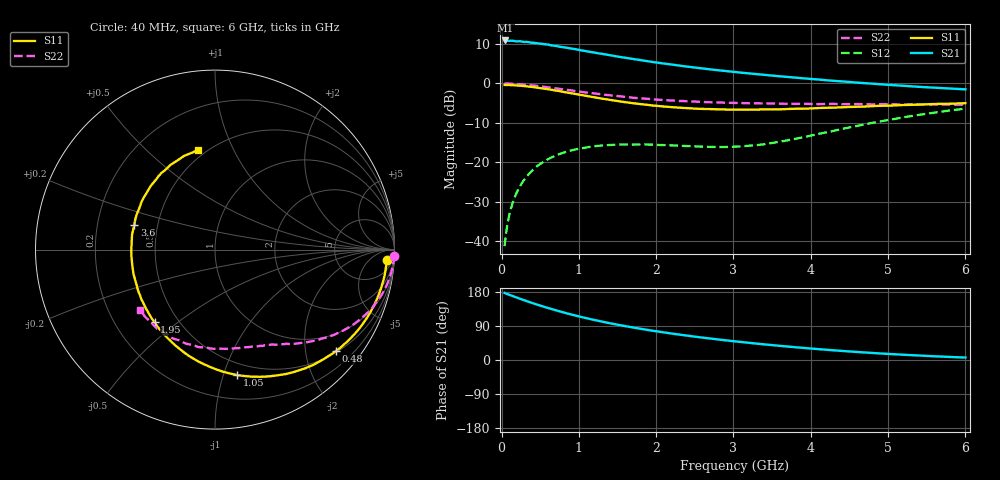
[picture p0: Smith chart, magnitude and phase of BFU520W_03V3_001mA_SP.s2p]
! Filename:  P:\Prog\Test\Noise\ATS_data\Testdata_Net\Run2\BFU520W_APM2013_06_A05_03p3V_001mA_SP_CM01_D.s2p
! Date/Time: Tue 26/Mar/2013 18:01:38
! BFU520W_APM2013_06_A05_03p3V_1to20mA_SP_CM01_Bias1_R.s2p
! MDIF S-parameter v. bias file
! BFU520W_APM2013_06_A05_03p3V_1to20mA_SP_CM01
! Date/time Tue Mar 19 16:47:37 2013
! bias mode 1
! bias variable = I_out
! VAR bias_var= 1
! VAR V_out= 3.3000
! VAR I_out= 1.0000
! VAR V_in= 0.7950
! VAR I_in= 0.0111
! Device data file deembeded for feedlines and parallel
! Original file: \Run2\BFU520W_APM2013_06_A05_03p3V_001mA_SP_CM01_R.s2p
! Feed-files: PR019V01_070313_Feed1.s2p, PR019V01_070313_Feed2.s2p
! Parallel-file: PR019V01_070313_Par.s2p
# MHz S MA R 50
!  Freq-MHz  S11-mag  S11-arg  S21-mag  S21-arg  S12-mag  S12-arg  S22-mag  S22-arg
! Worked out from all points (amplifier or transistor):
!   98 points, 40 MHz to 6 GHz, reference 50 ohm
!   highest |S21| = 10.9 dB at 50 MHz (marker M1)
!   |S21| within 3 dB of that: start of sweep to 1.178 GHz
!   unconditionally stable (mu >= 1): 2.745 GHz to 3.853 GHz
!   at 300 MHz: K = 0.12, MSG = 17.4 dB, |S12| = -24.2 dB
!   at 1.6 GHz: K = 0.58, MSG = 11.0 dB, |S12| = -15.5 dB
!   at 6 GHz: K = 0.83, MSG = 2.4 dB, |S12| = -6.4 dB
!   S11 on the Smith chart (normalised r, x): 40 MHz: 15, -22; 480 MHz: 0.53, -2.66; 1.05 GHz: 0.39, -1.11; 1.95 GHz: 0.37, -0.42; 3.6 GHz: 0.37, +0.13; 6 GHz: 0.45, +0.73
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40  0.9588 -3.5  3.496 177.0  0.008681 87.4  0.9983 -1.9
50  0.9588 -4.3  3.506 176.2  0.01076 87.0  0.9974 -2.3
100  0.9558 -8.6  3.46 172.1  0.02143 84.1  0.9949 -4.9
120  0.9533 -10.4  3.484 170.6  0.02562 82.9  0.9937 -5.8
200  0.9434 -17.1  3.414 164.6  0.04216 78.5  0.9841 -9.6
240  0.9362 -20.5  3.428 161.6  0.05004 76.4  0.9777 -11.5
340  0.9162 -28.8  3.35 154.4  0.06885 71.3  0.9579 -15.9
480  0.8797 -39.9  3.2 144.9  0.09247 64.5  0.9257 -21.7
600  0.8454 -49.2  3.114 137.3  0.1097 59.3  0.8936 -26.1
700  0.8138 -56.6  2.995 131.3  0.122 55.3  0.8671 -29.6
850  0.7671 -67.1  2.828 122.8  0.1373 50.0  0.8281 -34.1
1050  0.7093 -80.1  2.609 112.7  0.1518 44.1  0.778 -39.5
1250  0.6551 -92.3  2.413 103.5  0.1622 39.2  0.738 -44.0
1500  0.5993 -106.5  2.195 93.1  0.1681 34.5  0.6924 -49.2
1950  0.5261 -129.7  1.874 77.4  0.1677 30.1  0.6317 -57.0
2050  0.5161 -134.5  1.815 74.4  0.1661 29.9  0.6204 -58.5
2500  0.4797 -155.1  1.592 61.6  0.1596 31.3  0.59 -65.9
3100  0.4666 -179.4  1.37 47.5  0.1595 42.0  0.5649 -76.2
3600  0.4702 162.8  1.232 37.3  0.1828 52.4  0.5541 -85.5
4100  0.4884 147.0  1.121 28.6  0.2295 58.3  0.5476 -95.9
5200  0.5334 117.5  0.9349 13.8  0.3724 55.0  0.5404 -120.9
6000  0.5623 100.0  0.8426 6.4  0.4797 46.1  0.5357 -141.3
